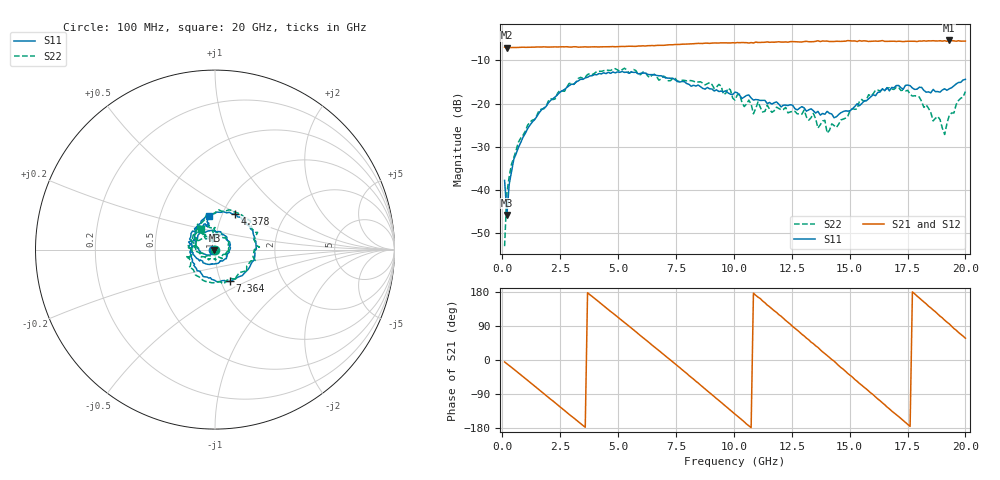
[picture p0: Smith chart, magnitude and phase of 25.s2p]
!Agilent Technologies,N5230C,MY49001569,A.09.33.09
!Agilent N5230C: A.09.33.09
!Date: Monday, July 27, 2015 10:25:50
!Correction: S11(Full 2 Port(1,2))
!S21(Full 2 Port(1,2))
!S12(Full 2 Port(1,2))
!S22(Full 2 Port(1,2))
!S2P File: Measurements: S11, S21, S12, S22:
# Hz S  dB  R 50
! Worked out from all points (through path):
!   201 points, 100 MHz to 20 GHz, reference 50 ohm
!   highest |S21| = -5.38 dB at 19.3 GHz (marker M1); lowest = -7.0 dB at 199.5 MHz (marker M2)
!   group delay of S21, straight-line fit = 142 ps
!   lowest |S11| = -45.8 dB at 199.5 MHz (marker M3), VSWR 1.01, Z = 49.7 - j0.404 ohm
!   |S11| at or under -10 dB: start of sweep to end of sweep
!   |S22| runs from -53.0 to -11.8 dB; largest |S21 - S12| = 0.022
!   S11 on the Smith chart (normalised r, x): 100 MHz: 0.97, -0.00; 4.378 GHz: 1.15, +0.48; 7.364 GHz: 1.11, -0.41; 20 GHz: 0.88, +0.34
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1e8  -37.80 -175.0  -6.96 -5.1  -6.94 -5.1  -53.05 -103.0
1.995e8  -45.81 -127.5  -7.05 -9.9  -7.02 -9.9  -40.63 -78.4
4.98e8  -32.90 -112.3  -7.00 -24.3  -7.05 -24.2  -32.52 -106.5
1.095e9  -25.81 -143.3  -6.96 -53.8  -6.96 -54.1  -25.00 -141.3
2.1895e9  -18.87 163.4  -6.87 -108.1  -6.87 -108.5  -19.08 164.1
3.483e9  -14.39 98.8  -6.91 -172.8  -6.91 -173.2  -14.16 98.0
4.3785e9  -12.86 60.5  -6.85 143.3  -6.91 142.7  -12.38 57.6
5.473e9  -12.97 14.5  -6.72 89.1  -6.71 88.7  -12.95 14.0
6.7665e9  -13.56 -38.1  -6.50 24.7  -6.49 24.2  -14.60 -43.3
7.3635e9  -14.14 -64.5  -6.38 -5.2  -6.38 -5.5  -14.17 -74.7
8.856e9  -16.28 -130.6  -6.01 -81.6  -5.98 -82.1  -15.42 -144.1
1.005e10  -17.36 165.5  -5.95 -142.9  -5.91 -143.6  -19.19 154.6
1.204e10  -20.77 63.7  -5.76 115.5  -5.68 114.0  -21.45 36.4
1.3433e10  -21.66 -0.2  -5.67 43.2  -5.60 41.9  -22.29 -28.9
1.403e10  -21.82 -38.9  -5.52 11.9  -5.56 11.3  -26.84 -65.1
1.47265e10  -21.84 -95.3  -5.56 -24.4  -5.53 -25.6  -23.61 -120.6
1.5622e10  -19.44 -143.4  -5.46 -71.7  -5.61 -72.7  -19.49 -178.5
1.67165e10  -17.06 160.5  -5.61 -128.9  -5.49 -129.2  -16.36 134.9
1.801e10  -16.23 113.6  -5.51 163.8  -5.51 162.5  -18.50 93.3
1.91045e10  -16.59 106.2  -5.45 105.1  -5.58 104.4  -27.17 105.6
1.93035e10  -16.57 103.6  -5.38 95.3  -5.56 94.5  -22.73 123.3
2e10  -14.40 99.5  -5.53 57.6  -5.42 55.9  -17.22 124.3
